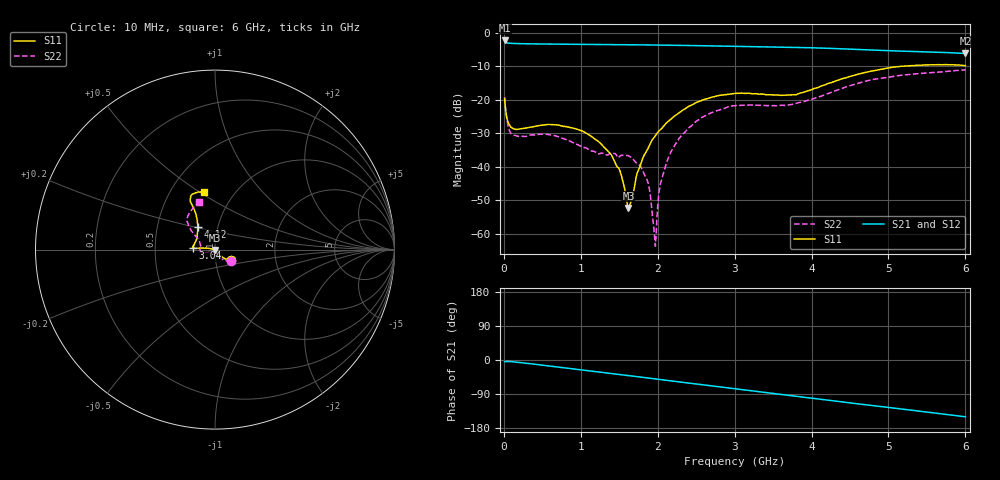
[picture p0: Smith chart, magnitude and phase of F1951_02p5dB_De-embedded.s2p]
! Integrated Device Technology
! Corporate Headquarters
! 6024 Silver Creek Valley Road
! San Jose, CA 95138  USA
! Phone:  1-408-284-8200
! Toll Free:  1-800-223-1366
! Webpage:  http://www.idt.com/
! Timing and RF Division
! 515 Groton Road, Suite 102
! Westford, MA 01886-6024
! Device:  F1951
! Description: 6-bit 0.5 dB Digital Step Attenuator
! Frequency:  100.0 -  4000.00 MHz
! Package:  4x4 mm Thin QFN Plastic Package: 24 pin
! Ports:  2 RF, 6 DC
!  Pin  1  = NC
!  Pin  2  = RF1  =  Port 1
!  Pin  3  = GND
!  Pin  4  = NC
!  Pin  5  = Serial Data Out (SDO)
!  Pin  6  = NC
!  Pin  7  = Reset Bar ( RSTb)
!  Pin  8  = Clock (CLK)
!  Pin  9  = Chip Select Bar (CSb)
!  Pin 10  = NC
!  Pin 11  = Serial Data In (SDI)
!  Pin 12  = NC
!  Pin 13  = NC
!  Pin 14  = VDD
!  Pin 15  = NC
!  Pin 16  = GND
!  Pin 17  = RF2  =  Port 2
!  Pin 18  = NC
!  Pin 19  = GND
!  Pin 20  = GND
!  Pin 21  = GND
!  Pin 22  = GND
!  Pin 23  = GND
!  Pin 24  = GND
! State:  5
! Atten State:  2.5 dB
! Voltage:  +3.30 Volts
! Current:  0.488 mA
! Data:  The device was measured on a F195X evaluation board which has
!  individual transmission lines to the RF pins.  Data was collected
!  de-embedded using a Automatic Fixture Removal [AFR] (Keysight Technologies).
!  The reference plane is the edge of the package pin.
! Misc:  Lot Code  1225BCA
!  Action Tracker AT0399
! Date Measured:  2018-09-13
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# GHz S dB R 50
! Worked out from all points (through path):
!   600 points, 10 MHz to 6 GHz, reference 50 ohm
!   highest |S21| = -2.28 dB at 10 MHz (marker M1); lowest = -6.2 dB at 6 GHz (marker M2)
!   group delay of S21, straight-line fit = 68.9 ps
!   lowest |S11| = -52.2 dB at 1.62 GHz (marker M3), VSWR 1.00, Z = 49.9 - j0.228 ohm
!   |S11| at or under -10 dB: start of sweep to 5.158 GHz
!   |S22| runs from -63.6 to -11.1 dB; largest |S21 - S12| = 0.00084
!   S11 on the Smith chart (normalised r, x): 10 MHz: 1.19, -0.13; 3.04 GHz: 0.78, +0.01; 4.12 GHz: 0.80, +0.21; 6 GHz: 0.73, +0.52
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0.01  -19.63 -32.2  -2.28 -4.6  -2.29 -4.6  -19.13 -35.6
0.07  -27.30 -49.3  -3.10 -3.9  -3.10 -4.0  -28.97 -62.3
0.12  -28.55 -54.7  -3.17 -4.8  -3.17 -4.8  -30.43 -67.2
0.64  -27.41 -76.1  -3.37 -17.0  -3.37 -17.0  -30.54 -80.1
1.01  -29.20 -67.1  -3.45 -26.0  -3.46 -26.0  -33.93 -55.5
1.4  -36.52 -54.0  -3.51 -35.6  -3.51 -35.6  -35.91 -2.8
1.52  -41.94 -54.2  -3.54 -38.4  -3.54 -38.4  -36.62 11.8
1.62  -52.20 -111.7  -3.55 -41.0  -3.56 -41.0  -36.67 14.6
1.86  -35.16 169.7  -3.61 -47.1  -3.61 -47.1  -43.74 16.0
1.96  -31.02 168.1  -3.64 -49.7  -3.64 -49.7  -61.00 -56.9
1.98  -30.37 168.2  -3.64 -50.2  -3.64 -50.2  -60.01 -141.8
2.01  -29.43 169.6  -3.65 -50.9  -3.65 -50.9  -49.05 -156.9
2.04  -28.78 170.0  -3.66 -51.7  -3.66 -51.7  -44.62 -152.2
2.12  -26.72 170.7  -3.69 -53.7  -3.69 -53.7  -38.40 -156.7
2.29  -23.62 172.6  -3.74 -58.0  -3.75 -58.1  -31.17 -159.8
2.6  -19.91 175.7  -3.87 -65.9  -3.87 -65.9  -24.92 -163.6
3.01  -18.06 176.5  -4.04 -76.0  -4.04 -76.0  -21.70 -172.4
3.04  -18.06 176.1  -4.05 -76.7  -4.06 -76.7  -21.69 -173.1
4.01  -16.86 132.0  -4.47 -101.2  -4.47 -101.1  -19.78 150.9
4.12  -15.91 127.0  -4.55 -103.9  -4.55 -103.9  -18.94 148.0
5.01  -10.45 117.1  -5.35 -125.3  -5.36 -125.3  -13.25 135.0
6  -9.76 101.2  -6.16 -149.9  -6.17 -149.9  -11.05 108.5
